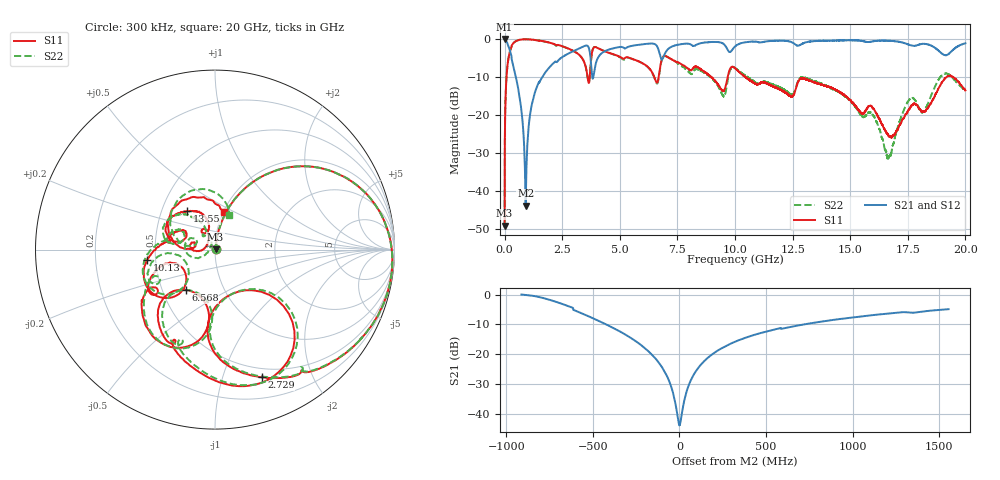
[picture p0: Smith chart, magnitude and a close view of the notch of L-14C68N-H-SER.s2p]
!{L-14C68N}
!Johanson Technology Inc.
!www.johansontechnology.com
!Test Board Conditions:
!Substrate Type  RO4350B
!Substrate Thickness  20 mil
!Substrate Dk  3.66
!TL Type: GCPW
!TL Trace Width  36 mil
!TL Gap  12 mil
!Electrode orientation  Horizontal
!DUT TOPOLOGY	SERIES
!Mounting Pad LxW  26x36 mil
! Created Sun Jun 20 13:07:38 2021
# hz S ma R 50
! 2 Port Network Data from SP1.SP block
! freq  magS11  angS11  magS21  angS21  magS12  angS12  magS22  angS22
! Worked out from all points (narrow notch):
!   20001 points, 300 kHz to 20 GHz, reference 50 ohm
!   highest |S21| = -0.01 dB at 1.3 MHz (marker M1); lowest = -43.8 dB at 913.3 MHz (marker M2)
!   notch at M2: 42.3 dB deep, 259 MHz wide at half that depth
!   lowest |S11| = -49.0 dB at 300 kHz (marker M3), VSWR 1.01, Z = 50.3 + j0.124 ohm
!   |S11| at or under -10 dB: 8.969 GHz to 9.682 GHz (712.8 MHz wide, 7.64 % of centre); 10.45 GHz to 19.18 GHz (8.728 GHz wide, 58.9 % of centre); 19.48 GHz to end of sweep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
!   |S22| runs from -49.6 to -0.1 dB; largest |S21 - S12| = 0.012
!   S11 on the Smith chart (normalised r, x): 300 kHz: 1.01, +0.00; 2.729 GHz: 0.40, -1.35; 6.568 GHz: 0.66, -0.32; 10.13 GHz: 0.45, -0.06; 13.55 GHz: 0.68, +0.31; 20 GHz: 1.01, +0.43
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300000  0.003533 20.5  0.9975 -0.2  0.9957 -0.1  0.003329 15.2
1300000  0.005507 73.2  0.9983 -0.3  0.9982 -0.4  0.005625 72.3
1.053e8  0.3895 63.4  0.9027 -24.1  0.9038 -24.0  0.3906 63.3
1.903e8  0.6108 48.5  0.7706 -39.7  0.7715 -39.7  0.6126 48.4
9.133e8  0.9929 -9.0  0.006488 -10.5  0.006635 -10.7  0.9928 -9.2
1.3993e9  0.9626 -28.2  0.2341 60.3  0.2349 60.1  0.9619 -28.2
2.7293e9  0.7576 -69.9  0.6353 19.1  0.6354 19.1  0.7573 -69.2
3.3343e9  0.5771 -90.1  0.7761 -3.1  0.7771 -3.2  0.5774 -88.6
3.8143e9  0.7099 -52.5  0.3056 -29.4  0.3056 -29.4  0.7106 -50.6
4.7743e9  0.621 -108.8  0.7616 -18.9  0.7634 -18.9  0.6196 -105.2
6.5683e9  0.278 -126.2  0.8386 -63.8  0.8394 -63.8  0.2725 -124.4
6.6673e9  0.2901 -102.9  0.7447 -70.4  0.7446 -70.2  0.2822 -100.6
7.0073e9  0.5951 -125.3  0.683 -47.2  0.6837 -47.1  0.593 -123.4
9.4973e9  0.2072 -145.9  0.8656 -100.4  0.8677 -100.5  0.1769 -156.5
1.00003e10  0.4138 -163.3  0.7985 -91.0  0.7997 -90.9  0.416 -165.4
1.01273e10  0.3832 -171.4  0.8492 -93.5  0.8522 -93.6  0.3886 -173.3
1.33343e10  0.277 131.1  0.9315 -139.8  0.9289 -139.8  0.2864 137.7
1.35513e10  0.2633 125.9  0.9431 -143.4  0.9341 -143.0  0.2726 134.0
1.59533e10  0.1278 116.8  0.9295 -178.5  0.9298 -178.5  0.1037 119.6
1.66673e10  0.0536 138.9  0.9483 168.6  0.9486 168.8  0.0281 153.2
1.75873e10  0.1221 -178.3  0.8335 153.4  0.8353 153.4  0.1625 -176.8
2e10  0.2116 76.8  0.8795 140.9  0.8769 141.1  0.2074 67.5
